FUNCTION "Binäruntersetzer FC" : VOID
TITLE =Binaeruntersetzer
VERSION : 0.1

BEGIN
NETWORK
TITLE =Merker 1
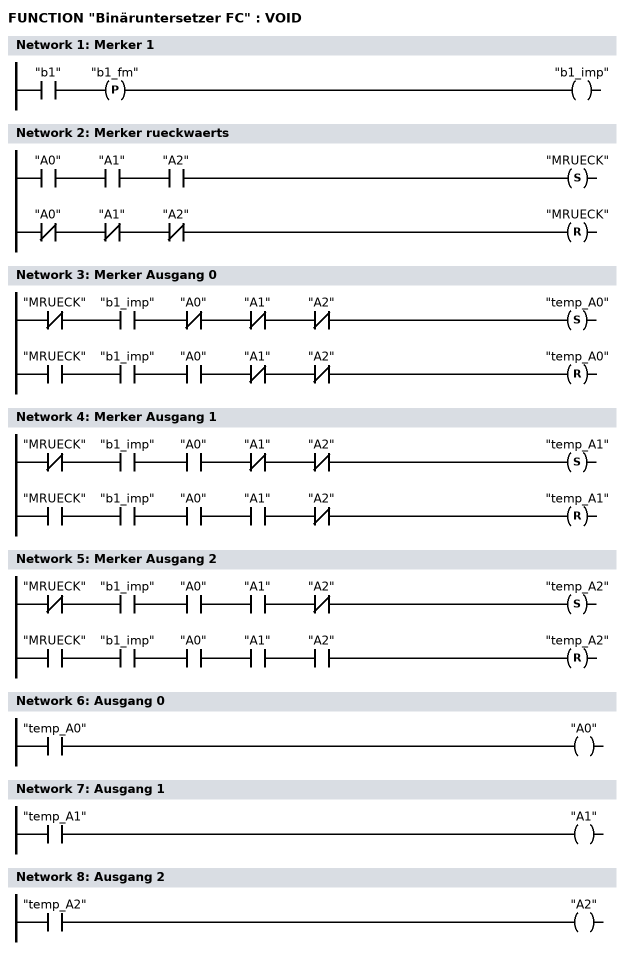
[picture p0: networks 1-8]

      U     "b1";
      FP    "b1_fm";
      =     "b1_imp";
NETWORK
TITLE =Merker rueckwaerts

      U     "A0";
      U     "A1";
      U     "A2";
      S     "MRUECK";
      UN    "A0";
      UN    "A1";
      UN    "A2";
      R     "MRUECK";
      NOP   0;
NETWORK
TITLE =Merker Ausgang 0

      UN    "MRUECK";
      U     "b1_imp";
      UN    "A0";
      UN    "A1";
      UN    "A2";
      S     "temp_A0";
      U     "MRUECK";
      U     "b1_imp";
      U     "A0";
      UN    "A1";
      UN    "A2";
      R     "temp_A0";
      NOP   0;
NETWORK
TITLE =Merker Ausgang 1

      UN    "MRUECK";
      U     "b1_imp";
      U     "A0";
      UN    "A1";
      UN    "A2";
      S     "temp_A1";
      U     "MRUECK";
      U     "b1_imp";
      U     "A0";
      U     "A1";
      UN    "A2";
      R     "temp_A1";
      NOP   0;
NETWORK
TITLE =Merker Ausgang 2

      UN    "MRUECK";
      U     "b1_imp";
      U     "A0";
      U     "A1";
      UN    "A2";
      S     "temp_A2";
      U     "MRUECK";
      U     "b1_imp";
      U     "A0";
      U     "A1";
      U     "A2";
      R     "temp_A2";
      NOP   0;
NETWORK
TITLE =Ausgang 0

      U     "temp_A0";
      =     "A0";
NETWORK
TITLE =Ausgang 1

      U     "temp_A1";
      =     "A1";
NETWORK
TITLE =Ausgang 2

      U     "temp_A2";
      =     "A2";
END_FUNCTION


ORGANIZATION_BLOCK "CYCLE"
BEGIN
	// Eingangssignal simulieren
	UN	M 16.0
	L	S5T#1S
	SE	T 1
	U	T 1
	=	M 16.0
	X	M 16.0
	X	M 16.1
	=	M 16.1
	=	"b1"

	// Binaeruntersetzer aufrufen
	CALL	FC 4
END_ORGANIZATION_BLOCK
